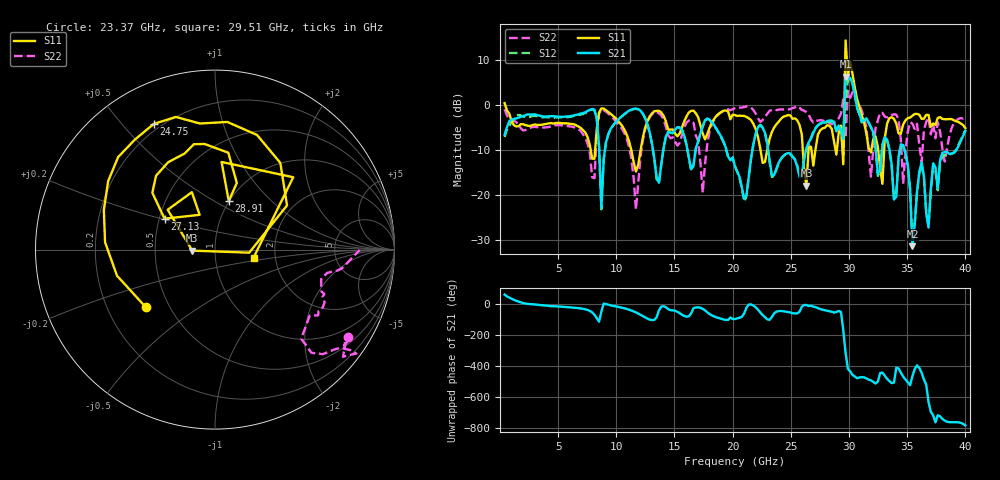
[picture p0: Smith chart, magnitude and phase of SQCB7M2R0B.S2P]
! Network Analyzer HP8722ES.07.66: Jul 25, 2000 Serial No. US39175408
! 26 Oct 2004  12:48:39
! Frequency  S11  S21  S12  S22
# HZ  S  DB R  50
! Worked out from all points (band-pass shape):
!   201 points, 400 MHz to 40 GHz, reference 50 ohm
!   highest |S21| = 6.41 dB at 29.7 GHz (marker M1); lowest = -31.4 dB at 35.45 GHz (marker M2)
!   |S21| within 3 dB of the highest: 29.66 GHz to 30.42 GHz (758.4 MHz wide, 2.52 % of centre)
!   lowest |S11| = -17.9 dB at 26.34 GHz (marker M3), VSWR 1.29, Z = 38.8 - j0.449 ohm
!   |S11| at or under -10 dB: 7.8 GHz to 8.179 GHz (379.3 MHz wide, 4.75 % of centre); 11.29 GHz to 12.09 GHz (797.2 MHz wide, 6.82 % of centre); 22.39 GHz to 22.97 GHz (579.9 MHz wide, 2.56 % of centre)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
!   |S22| runs from -23.3 to 3.2 dB; largest |S21 - S12| = 1.7
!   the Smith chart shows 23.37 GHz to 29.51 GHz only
!   S11 on the Smith chart (normalised r, x): 23.37 GHz: 0.37, -0.32; 24.75 GHz: 0.17, +0.61; 27.13 GHz: 0.53, +0.21; 28.91 GHz: 0.99, +0.58; 29.51 GHz: 1.54, -0.14
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4e8  0.48 -31.3  -6.56 59.5  -7.09 65.1  -0.88 -23.1
7.132e9  -5.53 -100.0  -1.75 -31.8  -1.97 -32.7  -6.44 -141.8
8.716e9  -0.70 -54.6  -22.88 -49.6  -23.22 -43.1  -0.88 -74.6
1.1686e10  -14.79 -48.7  -0.76 -55.3  -0.82 -55.9  -23.27 117.8
1.3666e10  -1.25 -35.0  -17.30 -42.2  -17.32 -40.3  -1.81 -73.7
2.02e10  -2.19 -31.4  -13.69 -98.0  -13.62 -98.6  -0.65 -27.1
2.3368e10  -5.99 -140.3  -15.69 -84.8  -15.98 -84.4  -1.05 -33.5
2.4754e10  -2.17 116.0  -10.69 -53.1  -10.88 -52.9  -0.95 -36.2
2.6338e10  -17.95 -177.4  -9.57 -8.1  -9.81 -9.4  -1.54 -44.1
2.6932e10  -13.48 113.8  -6.17 -18.1  -5.83 -19.5  -3.83 -34.9
2.713e10  -9.64 148.5  -5.09 -21.6  -5.03 -22.4  -3.33 -32.5
2.8912e10  -11.02 74.2  -5.80 -52.2  -5.81 -51.8  -3.18 -9.7
2.9506e10  -13.17 -11.7  -7.50 -170.2  -11.16 -62.5  1.45 33.0
2.9704e10  14.47 81.9  6.41 44.8  0.75 97.4  -7.25 -46.9
2.9902e10  6.50 -110.3  5.81 -57.6  5.66 -57.4  3.22 -19.7
3.01e10  9.74 -142.7  6.13 -74.1  5.91 -76.2  1.66 -26.3
3.0496e10  3.99 173.1  2.51 -106.7  2.30 -107.4  1.91 -60.2
3.0694e10  1.37 -32.9  -0.57 -118.2  -0.68 -119.3  0.46 111.1
3.1486e10  -6.21 136.4  -2.90 -119.0  -3.00 -119.6  -4.85 -105.3
3.3466e10  -2.89 -128.7  -9.76 -136.2  -10.03 -134.8  -2.66 -11.7
3.5446e10  -2.33 -145.5  -31.45 -105.8  -30.29 -107.9  -4.10 5.3
4e10  -5.10 -159.6  -5.72 -61.2  -5.54 -61.5  -2.54 66.4
